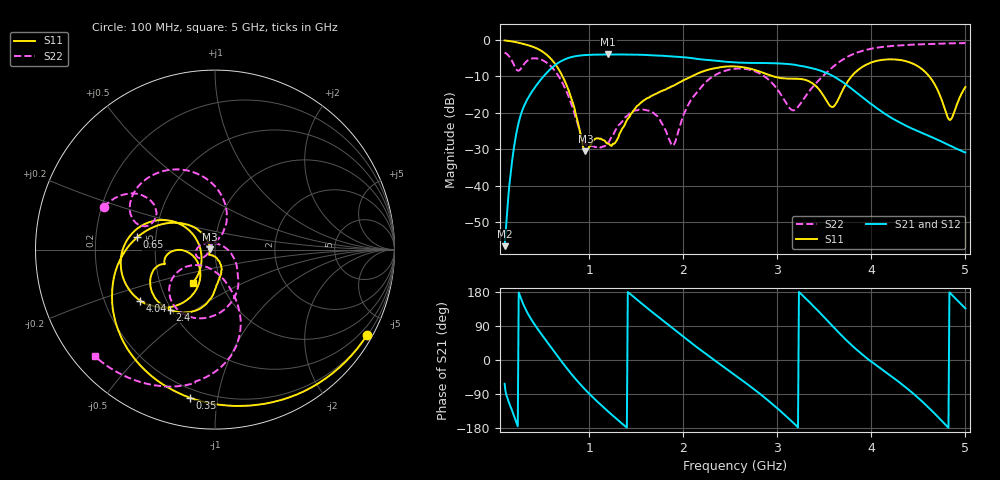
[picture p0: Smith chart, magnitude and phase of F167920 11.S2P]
!  2-Port S-parameters saved by WinCal
! VAR MeasName=S-Parameters (CALIBRATED_DATA) read from VNA (N5242A)
! VAR MeasDate=2016-11-22 9:54:07
! VAR NAME=F167920 11
! VAR FILENAME=F167920 11.S2P
! VAR DATE=2016-11-22 9:54:08
! VAR PHYS_PORTS=1,2
# Hz S DB R 50
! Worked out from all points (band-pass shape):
!   491 points, 100 MHz to 5 GHz, reference 50 ohm
!   highest |S21| = -4.08 dB at 1.2 GHz (marker M1); lowest = -56.6 dB at 100 MHz (marker M2)
!   |S21| within 3 dB of the highest: 633.1 MHz to 3.217 GHz (2.584 GHz wide, 134 % of centre)
!   lowest |S11| = -30.6 dB at 960 MHz (marker M3), VSWR 1.06, Z = 47.1 + j0.215 ohm
!   |S11| at or under -10 dB: 714.4 MHz to 2.094 GHz (1.38 GHz wide, 98.2 % of centre); 2.945 GHz to 3.792 GHz (847.1 MHz wide, 25.1 % of centre); 4.613 GHz to end of sweep
!   |S22| runs from -29.6 to -1.0 dB; largest |S21 - S12| = 0.0011
!   S11 on the Smith chart (normalised r, x): 100 MHz: 0.22, -3.82; 350 MHz: 0.15, -0.83; 650 MHz: 0.39, +0.07; 2.4 GHz: 0.49, -0.40; 4.04 GHz: 0.36, -0.27; 5 GHz: 0.73, -0.29
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1e8  -0.25 -29.3  -56.63 -62.9  -56.74 -65.3  -3.57 159.1
2.1e8  -0.66 -60.7  -27.87 -154.2  -27.85 -154.1  -7.49 143.6
3.5e8  -1.55 -99.7  -16.00 121.3  -16.00 121.4  -5.64 155.3
5e8  -3.25 -143.4  -10.51 65.1  -10.50 65.1  -5.62 123.2
6.5e8  -7.16 171.0  -6.75 14.5  -6.74 14.5  -9.11 89.7
9.2e8  -27.53 138.3  -4.31 -68.2  -4.31 -68.2  -26.97 85.7
9.6e8  -30.58 175.6  -4.24 -78.9  -4.24 -78.9  -28.67 106.6
1.2e9  -28.50 -123.1  -4.08 -135.8  -4.08 -135.8  -28.25 -165.5
1.46e9  -19.85 -70.0  -4.15 169.2  -4.15 169.2  -19.76 -153.6
1.74e9  -14.47 -86.0  -4.40 112.7  -4.40 112.6  -21.56 161.8
1.9e9  -12.59 -91.1  -4.65 81.1  -4.64 81.1  -28.83 57.8
2.4e9  -7.55 -127.1  -5.95 -12.9  -5.94 -13.0  -8.97 -86.8
2.55e9  -7.35 -141.2  -6.26 -39.8  -6.26 -39.9  -8.00 -107.2
2.92e9  -9.77 -164.5  -6.45 -110.5  -6.45 -110.6  -11.29 -147.3
3.16e9  -10.69 -164.3  -6.83 -163.3  -6.83 -163.4  -19.36 -116.9
3.37e9  -11.92 -176.2  -7.85 145.7  -7.85 145.7  -13.17 -69.4
3.59e9  -18.48 -146.3  -9.97 88.9  -9.96 88.9  -7.54 -70.1
4.04e9  -5.95 -145.5  -18.46 -11.6  -18.47 -11.8  -2.31 -101.2
4.19e9  -5.43 -162.6  -21.10 -39.0  -21.10 -39.1  -1.82 -109.8
4.58e9  -9.06 152.2  -26.06 -118.6  -26.08 -118.7  -1.24 -126.1
4.83e9  -21.99 -174.9  -28.99 178.4  -29.00 178.8  -1.05 -133.8
5e9  -13.00 -123.8  -30.94 136.1  -31.02 136.0  -0.97 -138.4
